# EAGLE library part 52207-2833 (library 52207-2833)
FFC & FPC Connectors 1.0 FPC ZIF 28Ckt Sn-Ag-Bi Source: Datasheet
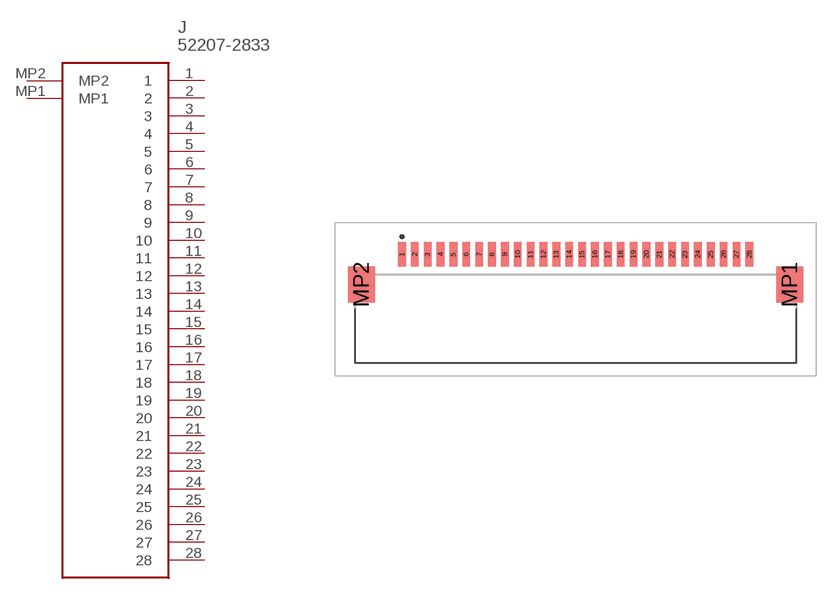
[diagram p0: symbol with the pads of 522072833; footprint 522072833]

Designator prefix J

## 52207-2833 (Description: FFC & FPC Connectors 1.0 FPC ZIF 28Ckt Sn-Ag-Bi; Height: 2.9mm; Manufacturer_Name: Molex; Manufacturer_Part_Number: 52207-2833; Mouser_Part_Number: 538-52207-2833; Mouser_Price-Stock: https://www.mouser.co.uk/ProductDetail/Molex/52207-2833?qs=rw2VfpiI%2FsNYNKizVECc7g%3D%3D)  [522072833]
1  1
2  2
3  3
4  4
5  5
6  6
7  7
8  8
9  9
10  10
11  11
12  12
13  13
14  14
15  15
16  16
17  17
18  18
19  19
20  20
21  21
22  22
23  23
24  24
25  25
26  26
27  27
28  28
MP1  MP1
MP2  MP2

## Footprint 522072833 (pad centres in mm)
52207-2833-1
smd 0.6 x 1.9: 1 -13.5,4.225; 2 -12.5,4.225; 3 -11.5,4.225; 4 -10.5,4.225; 5 -9.5,4.225; 6 -8.5,4.225; 7 -7.5,4.225; 8 -6.5,4.225; 9 -5.5,4.225; 10 -4.5,4.225; 11 -3.5,4.225; 12 -2.5,4.225; 13 -1.5,4.225; 14 -0.5,4.225; 15 0.5,4.225; 16 1.5,4.225; 17 2.5,4.225; 18 3.5,4.225; 19 4.5,4.225; 20 5.5,4.225; 21 6.5,4.225; 22 7.5,4.225; 23 8.5,4.225; 24 9.5,4.225; 25 10.5,4.225; 26 11.5,4.225; 27 12.5,4.225; 28 13.5,4.225
smd 2.1 x 2.8: MP1 16.65,1.875; MP2 -16.65,1.875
